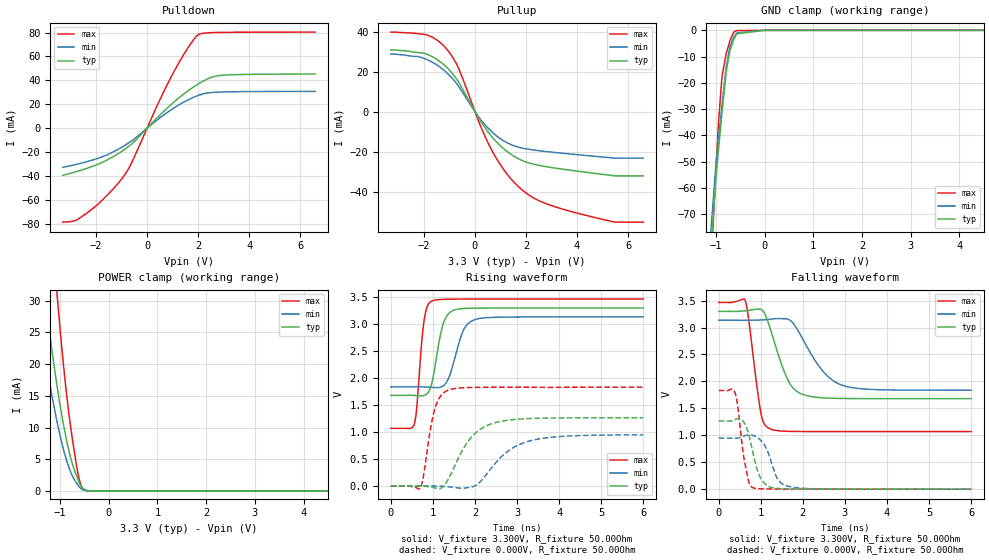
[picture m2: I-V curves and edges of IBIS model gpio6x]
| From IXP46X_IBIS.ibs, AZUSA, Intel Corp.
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[Model]   gpio6x
Model_type   I/O
Vinl = 800.000mV
Vinh = 2.000V
Vmeas = 1.500V
Cref = 0.000F
|   typ   min   max
C_comp   1.100pF   0.800pF   2.000pF
[Voltage Range]   3.300V   3.135V   3.465V
[Temperature Range]   25.0   110.0   -40.0
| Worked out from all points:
|   slope of the pulldown table from 0 to 0.495 V, typ, clamps not added: 45.9 ohm
|   slope of the pullup table from 0 to 0.495 V, typ, clamps not added: 50.2 ohm
|   POWER clamp passes 1 mA (typ) near -0.59 V on its own axis
|   falling waveform, V_fixture 3.300V, R_fixture 50.00Ohm: 20-80 % time 434ps typ, 655ps min, 234ps max; typ from 3.3 V to 1.68 V
|   rising waveform, V_fixture 3.300V, R_fixture 50.00Ohm: 20-80 % time 232ps typ, 300ps min, 150ps max; typ from 1.68 V to 3.3 V
|   rising waveform, V_fixture 0.000V, R_fixture 50.00Ohm: 20-80 % time 610ps typ, 781ps min, 249ps max; typ from 0 V to 1.27 V
|   falling waveform, V_fixture 0.000V, R_fixture 50.00Ohm: 20-80 % time 252ps typ, 272ps min, 187ps max; typ from 1.27 V to 0 V
[Pulldown]
|   Voltage   I(typ)   I(min)   I(max)
-3.3V     -39.35mA   -32.68mA   -78.59mA
-2.8V     -36.5mA    -30.4mA    -77.05mA
-2.28V    -32.98mA   -27.52mA   -69.69mA
-1.61V    -27.01mA   -22.68mA   -57.04mA
-935mV    -18.57mA   -15.21mA   -40.69mA
-605mV    -13.24mA   -10.63mA   -28.92mA
940mV     19.72mA    15.35mA    42.71mA
1.535V    30.16mA    22.95mA    64.94mA
1.99V     36.76mA    27.28mA    77.99mA
2.545V    42.79mA    29.85mA    79.92mA
2.875V    44.1mA     30.23mA    80.1mA
6.595V    45.33mA    30.81mA    80.37mA
[GND Clamp]
|   Voltage   I(typ)   I(min)   I(max)
-3.3V     -1.837A    -1.782A    -2.189A
-1.11V    -84.97mA   -78.05mA   -94.05mA
-1V       -56.67mA   -51.68mA   -53.31mA
-945mV    -45.22mA   -41.04mA   -35.09mA
-875mV    -31.66mA   -28.71mA   -17.73mA
-790mV    -16.31mA   -14.35mA   -9.037mA
-785mV    -15.46mA   -13.74mA   -8.626mA
-710mV    -7.709mA   -6.046mA   -3.931mA
-635mV    -3.524mA   -2.728mA   -731.7uA
-575mV    -1.508mA   -1.11mA    -135.3uA
0V        -56.84nA   -17.58nA   -162.8pA
6.595V    0A         0A         0A
[Pullup]
|   Voltage   I(typ)   I(min)   I(max)
-3.3V     30.82mA    28.74mA    39.72mA
-1.9V     28.73mA    26.06mA    38.37mA
-1.065V   21.56mA    18.92mA    30.55mA
-630mV    14.5mA     12.45mA    21.24mA
215mV     -4.652mA   -3.833mA   -7.123mA
695mV     -13.05mA   -10.51mA   -20.13mA
1.25V     -19.87mA   -15.5mA    -31.1mA
1.945V    -24.91mA   -18.47mA   -40.12mA
2.53V     -26.9mA    -19.56mA   -44.63mA
3.775V    -29.37mA   -21.23mA   -49.98mA
5.5V      -32.12mA   -23.24mA   -55.25mA
6.595V    -32.12mA   -23.24mA   -55.25mA
[POWER Clamp]
|   Voltage   I(typ)   I(min)   I(max)
-3.3V     221.1mA    178.2mA    360.9mA
-1.505V   44.69mA    32.21mA    80.57mA
-1.435V   39.57mA    28.24mA    71.76mA
-1.33V    32.34mA    22.7mA     59.18mA
-1.265V   28.14mA    19.51mA    51.81mA
-1.085V   17.78mA    11.79mA    33.26mA
-1.025V   14.77mA    9.605mA    27.77mA
-880mV    8.535mA    5.208mA    16.26mA
-770mV    4.91mA     2.789mA    9.454mA
-640mV    1.999mA    1.036mA    3.043mA
-515mV    310.8uA    129.7uA    235.8uA
6.595V    0A         0A         0A
[Ramp]
R_load = 50.00Ohm
|   typ   min   max
dV/dt_r   759.567mV/608.821ps 569.138mV/780.708ps   1.099V/248.460ps
dV/dt_f   972.056mV/433.631ps 779.354mV/655.279ps   1.437V/233.958ps
[Falling Waveform]
V_fixture = 3.300V
V_fixture_min = 3.135V
V_fixture_max = 3.465V
R_fixture = 50.00Ohm
|   Time   V(typ)   V(min)   V(max)
0s        3.3V       3.135V     3.465V
630ps     3.31V      3.134V     3.499V
710ps     3.318V     3.135V     3.163V
1ns       3.339V     3.14V      1.422V
1.2ns     3.037V     3.152V     1.126V
1.64ns    2.033V     3.156V     1.074V
2.01ns    1.754V     2.768V     1.07V
2.5ns     1.694V     2.169V     1.069V
3ns       1.683V     1.913V     1.069V
6ns       1.68V      1.836V     1.069V
[Rising Waveform]
V_fixture = 3.300V
V_fixture_min = 3.135V
V_fixture_max = 3.465V
R_fixture = 50.00Ohm
|   Time   V(typ)   V(min)   V(max)
0s        1.68V      1.836V     1.069V
560ps     1.678V     1.837V     1.155V
610ps     1.676V     1.837V     1.401V
790ps     1.679V     1.836V     3.061V
960ps     1.867V     1.828V     3.423V
1.24ns    2.991V     1.854V     3.459V
1.51ns    3.263V     2.338V     3.464V
1.76ns    3.291V     2.935V     3.465V
2.1ns     3.297V     3.104V     3.465V
6ns       3.3V       3.135V     3.465V
[Rising Waveform]
V_fixture = 0.000V
V_fixture_min = 0.000V
V_fixture_max = 0.000V
R_fixture = 50.00Ohm
|   Time   V(typ)   V(min)   V(max)
0s        1.333uV    464.1nV    -6.996nV
700ps     -128.8uV   224.2uV    -42.38mV
770ps     -3.043mV   448uV      159.4mV
1.04ns    -34.26mV   190.8uV    1.412V
1.36ns    117.5mV    -13.64mV   1.774V
1.89ns    882.2mV    -23.51mV   1.826V
2.41ns    1.158V     352.6mV    1.831V
2.86ns    1.227V     686.7mV    1.831V
3.41ns    1.253V     856mV      1.83V
6ns       1.266V     948.6mV    1.832V
[Falling Waveform]
V_fixture = 0.000V
V_fixture_min = 0.000V
V_fixture_max = 0.000V
R_fixture = 50.00Ohm
|   Time   V(typ)   V(min)   V(max)
0s        1.266V     948.6mV    1.832V
390ps     1.289V     945mV      1.782V
620ps     1.212V     990.9mV    486mV
720ps     995mV      1.006V     123.4mV
820ps     652.4mV    995.4mV    24.75mV
960ps     263.3mV    932.9mV    9.268mV
1.1ns     99.15mV    802.3mV    5.623mV
1.39ns    14.72mV    204.3mV    1.559mV
1.65ns    5.303mV    53.87mV    322uV
6ns       1.333uV    464.1nV    -6.996nV
